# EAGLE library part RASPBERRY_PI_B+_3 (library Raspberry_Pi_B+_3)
Raspberry Pi, 2 B+ und 3
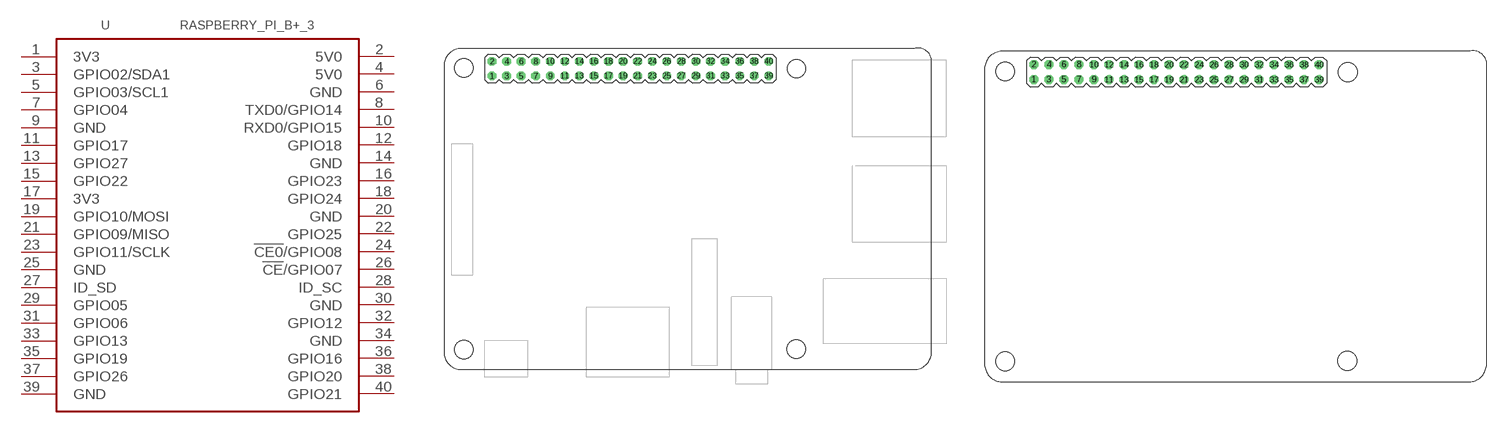
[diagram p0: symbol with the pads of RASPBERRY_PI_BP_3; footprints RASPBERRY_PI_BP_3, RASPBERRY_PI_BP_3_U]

Designator prefix -

## RASPBERRY_PI_B+_3_D  [RASPBERRY_PI_BP_3]
1  3V3  pwr
2  5V0  pwr
3  GPIO02/SDA1
4  5V0  pwr
5  GPIO03/SCL1
6  GND  pwr
7  GPIO04
8  TXD0/GPIO14
9  GND  pwr
10  RXD0/GPIO15
11  GPIO17
12  GPIO18
13  GPIO27
14  GND  pwr
15  GPIO22
16  GPIO23
17  3V3  pwr
18  GPIO24
19  GPIO10/MOSI
20  GND  pwr
21  GPIO09/MISO
22  GPIO25
23  GPIO11/SCLK
24  !CE0!/GPIO08
25  GND  pwr
26  !CE!/GPIO07
27  ID_SD
28  ID_SC
29  GPIO05
30  GND  pwr
31  GPIO06
32  GPIO12
33  GPIO13
34  GND  pwr
35  GPIO19
36  GPIO16
37  GPIO26
38  GPIO20
39  GND  pwr
40  GPIO21

## RASPBERRY_PI_B+_3_U  [RASPBERRY_PI_BP_3_U]
Pads as for RASPBERRY_PI_BP_3

## Footprint RASPBERRY_PI_BP_3 (pad centres in mm)
Raspberry Pi Board Version 2 B+ und 3
drill 1.016 octagon: 1 8.37,51.23; 2 8.37,53.77; 3 10.91,51.23; 4 10.91,53.77; 5 13.45,51.23; 6 13.45,53.77; 7 15.99,51.23; 8 15.99,53.77; 9 18.53,51.23; 10 18.53,53.77; 11 21.07,51.23; 12 21.07,53.77; 13 23.61,51.23; 14 23.61,53.77; 15 26.15,51.23; 16 26.15,53.77; 17 28.69,51.23; 18 28.69,53.77; 19 31.23,51.23; 20 31.23,53.77; 21 33.77,51.23; 22 33.77,53.77; 23 36.31,51.23; 24 36.31,53.77; 25 38.85,51.23; 26 38.85,53.77; 27 41.39,51.23; 28 41.39,53.77; 29 43.93,51.23; 30 43.93,53.77; 31 46.47,51.23; 32 46.47,53.77; 33 49.01,51.23; 34 49.01,53.77; 35 51.55,51.23; 36 51.55,53.77; 37 54.09,51.23; 38 54.09,53.77; 39 56.63,51.23; 40 56.63,53.77
hole 3.2 at 3.493,3.493
hole 3.2 at 61.469,52.482
hole 3.2 at 3.493,52.596
hole 3.2 at 61.437,3.524

## Footprint RASPBERRY_PI_BP_3_U (pad centres in mm)
Raspberry Pi Board Version 2 B+ und 3
drill 1.016 octagon: 1 8.37,51.23; 2 8.37,53.77; 3 10.91,51.23; 4 10.91,53.77; 5 13.45,51.23; 6 13.45,53.77; 7 15.99,51.23; 8 15.99,53.77; 9 18.53,51.23; 10 18.53,53.77; 11 21.07,51.23; 12 21.07,53.77; 13 23.61,51.23; 14 23.61,53.77; 15 26.15,51.23; 16 26.15,53.77; 17 28.69,51.23; 18 28.69,53.77; 19 31.23,51.23; 20 31.23,53.77; 21 33.77,51.23; 22 33.77,53.77; 23 36.31,51.23; 24 36.31,53.77; 25 38.85,51.23; 26 38.85,53.77; 27 41.39,51.23; 28 41.39,53.77; 29 43.93,51.23; 30 43.93,53.77; 31 46.47,51.23; 32 46.47,53.77; 33 49.01,51.23; 34 49.01,53.77; 35 51.55,51.23; 36 51.55,53.77; 37 54.09,51.23; 38 54.09,53.77; 39 56.63,51.23; 40 56.63,53.77
hole 3.2 at 3.493,3.493
hole 3.2 at 61.469,52.482
hole 3.2 at 3.493,52.596
hole 3.2 at 61.437,3.524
